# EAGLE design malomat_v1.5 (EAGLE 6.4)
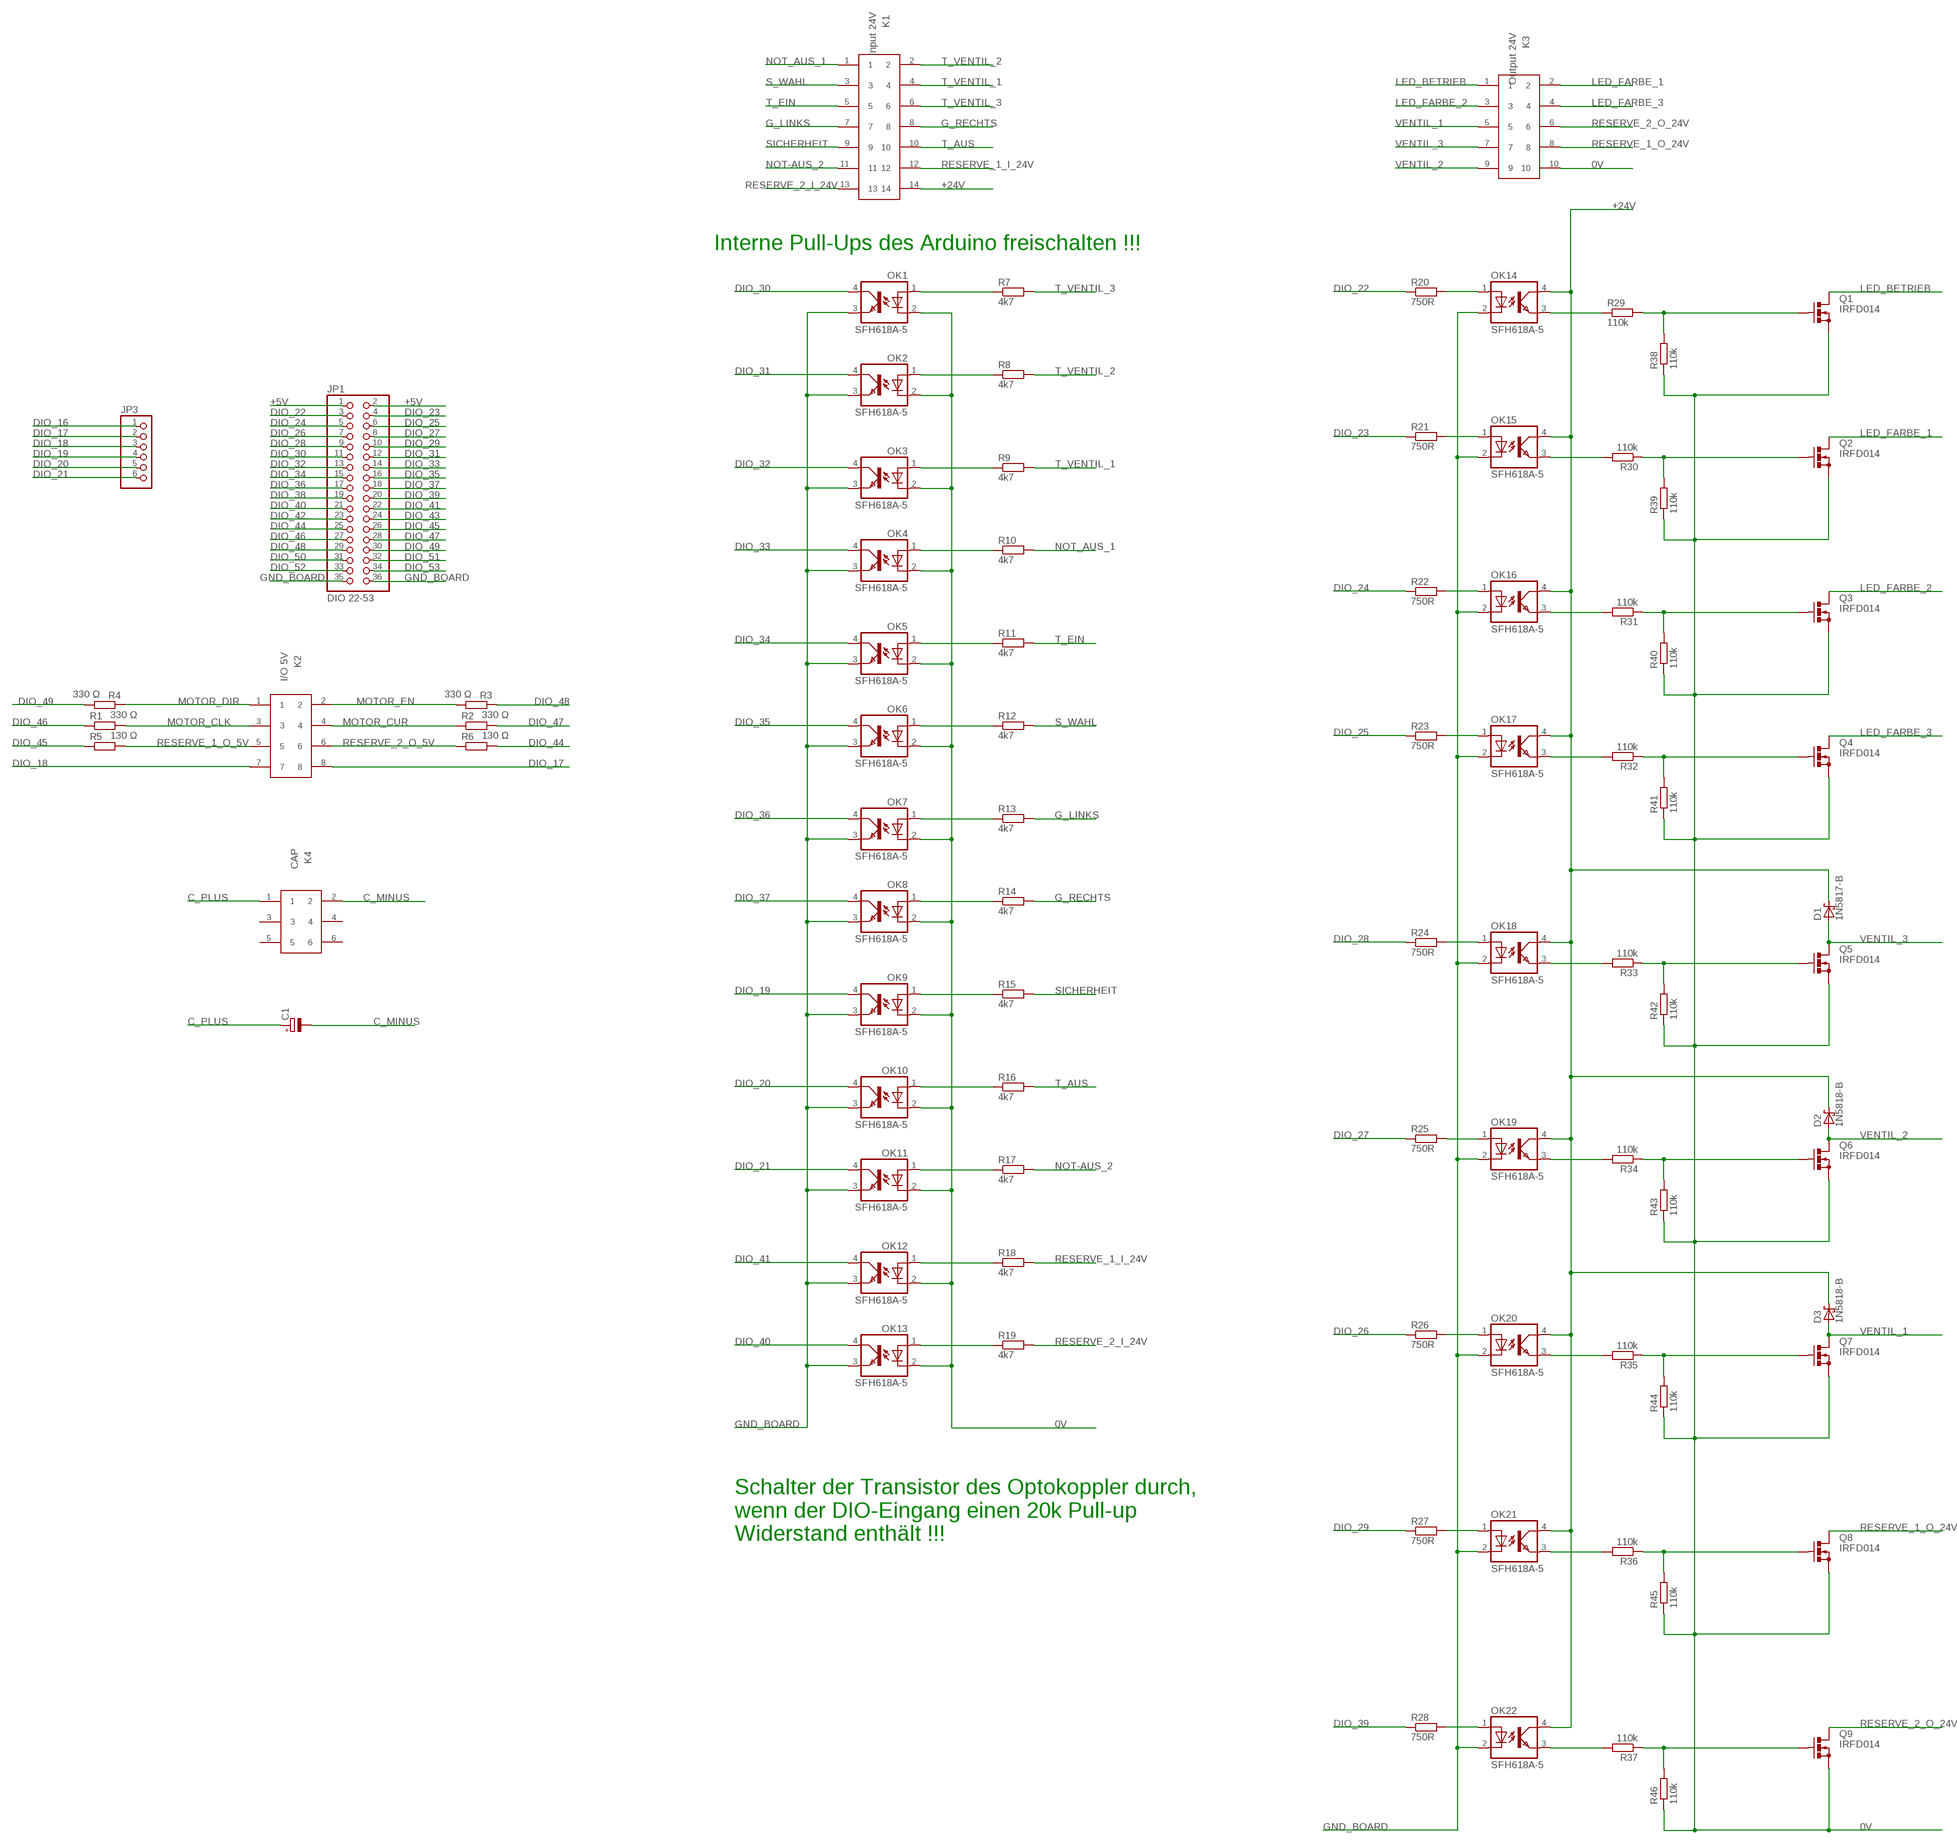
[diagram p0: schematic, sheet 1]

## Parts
C1  CPOL-EUE10-20  [EB20D]
D1  1N5817-B  [DO41-7.6]
D2  1N5818-B  [DO41-7.6]
D3  1N5818-B  [DO41-7.6]
JP1  DIO 22-53  PINHD-2X18  [2X18]
JP3  PINHD-1X6  [1X06]
K1  Input 24V  61201421621  [61201421621]
K2  I/O 5V  61200821621  [61200821621]
K3  Output 24V  61201021621  [61201021621]
K4  CAP  61200621621  [61200621621]
OK1  SFH618A-5  [DIP4]
OK2  SFH618A-5  [DIP4]
OK3  SFH618A-5  [DIP4]
OK4  SFH618A-5  [DIP4]
OK5  SFH618A-5  [DIP4]
OK6  SFH618A-5  [DIP4]
OK7  SFH618A-5  [DIP4]
OK8  SFH618A-5  [DIP4]
OK9  SFH618A-5  [DIP4]
OK10  SFH618A-5  [DIP4]
OK11  SFH618A-5  [DIP4]
OK12  SFH618A-5  [DIP4]
OK13  SFH618A-5  [DIP4]
OK14  SFH618A-5  [DIP4]
OK15  SFH618A-5  [DIP4]
OK16  SFH618A-5  [DIP4]
OK17  SFH618A-5  [DIP4]
OK18  SFH618A-5  [DIP4]
OK19  SFH618A-5  [DIP4]
OK20  SFH618A-5  [DIP4]
OK21  SFH618A-5  [DIP4]
OK22  SFH618A-5  [DIP4]
Q1  IRFD014  BS170  [C370-01]
Q2  IRFD014  BS170  [C370-01]
Q3  IRFD014  BS170  [C370-01]
Q4  IRFD014  BS170  [C370-01]
Q5  IRFD014  BS170  [C370-01]
Q6  IRFD014  BS170  [C370-01]
Q7  IRFD014  BS170  [C370-01]
Q8  IRFD014  BS170  [C370-01]
Q9  IRFD014  BS170  [C370-01]
R1  330 Ω  R-EU_0309/12  [0309/12]
R2  330 Ω  R-EU_0309/12  [0309/12]
R3  330 Ω  R-EU_0309/12  [0309/12]
R4  330 Ω  R-EU_0309/12  [0309/12]
R5  130 Ω  R-EU_0411/15  [0411/15]
R6  130 Ω  R-EU_0411/15  [0411/15]
R7  4k7  R-EU_0309/12  [0309/12]
R8  4k7  R-EU_0309/12  [0309/12]
R9  4k7  R-EU_0309/12  [0309/12]
R10  4k7  R-EU_0309/12  [0309/12]
R11  4k7  R-EU_0309/12  [0309/12]
R12  4k7  R-EU_0309/12  [0309/12]
R13  4k7  R-EU_0309/12  [0309/12]
R14  4k7  R-EU_0309/12  [0309/12]
R15  4k7  R-EU_0309/12  [0309/12]
R16  4k7  R-EU_0309/12  [0309/12]
R17  4k7  R-EU_0309/12  [0309/12]
R18  4k7  R-EU_0309/12  [0309/12]
R19  4k7  R-EU_0309/12  [0309/12]
R20  750R  R-EU_0204/7  [0204/7]
R21  750R  R-EU_0204/7  [0204/7]
R22  750R  R-EU_0204/7  [0204/7]
R23  750R  R-EU_0204/7  [0204/7]
R24  750R  R-EU_0204/7  [0204/7]
R25  750R  R-EU_0204/7  [0204/7]
R26  750R  R-EU_0204/7  [0204/7]
R27  750R  R-EU_0204/7  [0204/7]
R28  750R  R-EU_0204/7  [0204/7]
R29  110k  R-EU_0204/7  [0204/7]
R30  110k  R-EU_0204/7  [0204/7]
R31  110k  R-EU_0204/7  [0204/7]
R32  110k  R-EU_0204/7  [0204/7]
R33  110k  R-EU_0204/7  [0204/7]
R34  110k  R-EU_0204/7  [0204/7]
R35  110k  R-EU_0204/7  [0204/7]
R36  110k  R-EU_0204/7  [0204/7]
R37  110k  R-EU_0204/7  [0204/7]
R38  110k  R-EU_0204/7  [0204/7]
R39  110k  R-EU_0204/7  [0204/7]
R40  110k  R-EU_0204/7  [0204/7]
R41  110k  R-EU_0204/7  [0204/7]
R42  110k  R-EU_0204/7  [0204/7]
R43  110k  R-EU_0204/7  [0204/7]
R44  110k  R-EU_0204/7  [0204/7]
R45  110k  R-EU_0204/7  [0204/7]
R46  110k  R-EU_0204/7  [0204/7]

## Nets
0V: K3.10 OK1.2(C) OK2.2(C) OK3.2(C) OK4.2(C) OK5.2(C) OK6.2(C) OK7.2(C) OK8.2(C) OK9.2(C) OK10.2(C) OK11.2(C) OK12.2(C) OK13.2(C) Q1.S Q2.S Q3.S Q4.S Q5.S Q6.S Q7.S Q8.S Q9.S R38.1 R39.1 R40.1 R41.1 R42.1 R43.1 R44.1 R45.1 R46.1
+5V: JP1.1 JP1.2
+24V: D1.C D2.C D3.C K1.14 OK14.4(COL) OK15.4(COL) OK16.4(COL) OK17.4(COL) OK18.4(COL) OK19.4(COL) OK20.4(COL) OK21.4(COL) OK22.4(COL)
C_MINUS: C1.- K4.2
C_PLUS: C1.+ K4.1
DIO_16: JP3.1
DIO_17: JP3.2 K2.8
DIO_18: JP3.3 K2.7
DIO_19: JP3.4 OK9.4(COL)
DIO_20: JP3.5 OK10.4(COL)
DIO_21: JP3.6 OK11.4(COL)
DIO_22: JP1.3 R20.1
DIO_23: JP1.4 R21.1
DIO_24: JP1.5 R22.1
DIO_25: JP1.6 R23.1
DIO_26: JP1.7 R26.1
DIO_27: JP1.8 R25.1
DIO_28: JP1.9 R24.1
DIO_29: JP1.10 R27.1
DIO_30: JP1.11 OK1.4(COL)
DIO_31: JP1.12 OK2.4(COL)
DIO_32: JP1.13 OK3.4(COL)
DIO_33: JP1.14 OK4.4(COL)
DIO_34: JP1.15 OK5.4(COL)
DIO_35: JP1.16 OK6.4(COL)
DIO_36: JP1.17 OK7.4(COL)
DIO_37: JP1.18 OK8.4(COL)
DIO_38: JP1.19
DIO_39: JP1.20 R28.1
DIO_40: JP1.21 OK13.4(COL)
DIO_41: JP1.22 OK12.4(COL)
DIO_42: JP1.23
DIO_43: JP1.24
DIO_44: JP1.25 R6.2
DIO_45: JP1.26 R5.1
DIO_46: JP1.27 R1.1
DIO_47: JP1.28 R2.2
DIO_48: JP1.29 R3.1
DIO_49: JP1.30 R4.2
DIO_50: JP1.31
DIO_51: JP1.32
DIO_52: JP1.33
DIO_53: JP1.34
G_LINKS: K1.7 R13.2
G_RECHTS: K1.8 R14.2
GND_BOARD: JP1.35 JP1.36 OK1.3(EMIT) OK2.3(EMIT) OK3.3(EMIT) OK4.3(EMIT) OK5.3(EMIT) OK6.3(EMIT) OK7.3(EMIT) OK8.3(EMIT) OK9.3(EMIT) OK10.3(EMIT) OK11.3(EMIT) OK12.3(EMIT) OK13.3(EMIT) OK14.2(C) OK15.2(C) OK16.2(C) OK17.2(C) OK18.2(C) OK19.2(C) OK20.2(C) OK21.2(C) OK22.2(C)
LED_BETRIEB: K3.1 Q1.D
LED_FARBE_1: K3.2 Q2.D
LED_FARBE_2: K3.3 Q3.D
LED_FARBE_3: K3.4 Q4.D
MOTOR_CLK: K2.3 R1.2
MOTOR_CUR: K2.4 R2.1
MOTOR_DIR: K2.1 R4.1
MOTOR_EN: K2.2 R3.2
N$1: OK1.1(A) R7.1
N$2: OK2.1(A) R8.1
N$3: OK3.1(A) R9.1
N$4: OK22.1(A) R28.2
N$5: OK14.3(EMIT) R29.1
N$6: Q1.G R29.2 R38.2
N$7: OK4.1(A) R10.1
N$8: OK5.1(A) R11.1
N$9: OK6.1(A) R12.1
N$10: OK7.1(A) R13.1
N$13: OK21.1(A) R27.2
N$14: OK15.3(EMIT) R30.2
N$15: Q2.G R30.1 R39.2
N$16: OK8.1(A) R14.1
N$17: OK9.1(A) R15.1
N$18: OK10.1(A) R16.1
N$19: OK11.1(A) R17.1
N$20: OK12.1(A) R18.1
N$22: OK13.1(A) R19.1
N$23: OK20.1(A) R26.2
N$24: OK16.3(EMIT) R31.2
N$25: OK19.1(A) R25.2
N$26: Q3.G R31.1 R40.2
N$28: OK18.1(A) R24.2
N$29: OK17.1(A) R23.2
N$30: OK16.1(A) R22.2
N$31: OK15.1(A) R21.2
N$32: OK14.1(A) R20.2
N$35: OK17.3(EMIT) R32.2
N$36: Q4.G R32.1 R41.2
N$43: OK18.3(EMIT) R33.2
N$44: Q5.G R33.1 R42.2
N$50: OK19.3(EMIT) R34.2
N$51: Q6.G R34.1 R43.2
N$57: OK20.3(EMIT) R35.2
N$58: Q7.G R35.1 R44.2
N$64: OK21.3(EMIT) R36.2
N$65: Q8.G R36.1 R45.2
N$71: OK22.3(EMIT) R37.2
N$72: Q9.G R37.1 R46.2
NOT-AUS_2: K1.11 R17.2
NOT_AUS_1: K1.1 R10.2
RESERVE_1_I_24V: K1.12 R18.2
RESERVE_1_O_5V: K2.5 R5.2
RESERVE_1_O_24V: K3.8 Q8.D
RESERVE_2_I_24V: K1.13 R19.2
RESERVE_2_O_5V: K2.6 R6.1
RESERVE_2_O_24V: K3.6 Q9.D
S_WAHL: K1.3 R12.2
SICHERHEIT: K1.9 R15.2
T_AUS: K1.10 R16.2
T_EIN: K1.5 R11.2
T_VENTIL_1: K1.4 R9.2
T_VENTIL_2: K1.2 R8.2
T_VENTIL_3: K1.6 R7.2
VENTIL_1: D3.A K3.5 Q7.D
VENTIL_2: D2.A K3.9 Q6.D
VENTIL_3: D1.A K3.7 Q5.D
Unconnected: K4.3 K4.4 K4.5 K4.6

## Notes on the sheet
- Interne Pull-Ups des Arduino freischalten !!!
- Schalter der Transistor des Optokoppler durch, 
  wenn der DIO-Eingang einen 20k Pull-up 
  Widerstand enthält !!!

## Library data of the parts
C1 = resistor:CPOL-EU: POLARIZED CAPACITOR, European symbol
D1-D3 = diode:1N581*: 1.0A SCHOTTKY BARRIER RECTIFIER; MF: MULTICOMP; MPN: 1N4004; OC_FARNELL: 9565027
JP1 = pinhead:PINHD-2X18: PIN HEADER; MF: SAMTEC; MPN: TSW-118-07-F-D; OC_FARNELL: 2025187
JP3 = pinhead:PINHD-1X6: PIN HEADER
K1 = Wuerth_Elektronik_eiCan_05_Box_Header_IDC_Connectors_1_2:61201421621: WR-BHD 2.54mm Male Box Header, 14 Pins; MF: AMPHENOL; MPN: T821114A1R100CEU; OC_FARNELL: 2215292
K2 = Wuerth_Elektronik_eiCan_05_Box_Header_IDC_Connectors_1_2:61200821621: WR-BHD 2.54mm Male Box Header, 8 Pins; MF: AMPHENOL; MPN: T821108A1S100CEU; OC_FARNELL: 2215303
K3 = Wuerth_Elektronik_eiCan_05_Box_Header_IDC_Connectors_1_2:61201021621: WR-BHD 2.54mm Male Box Header, 10 Pins; MF: AMPHENOL; MPN: T821110A1S100CEU; OC_FARNELL: 2215304
K4 = Wuerth_Elektronik_eiCan_05_Box_Header_IDC_Connectors_1_2:61200621621: WR-BHD 2.54mm Male Box Header, 6 Pins
OK1-OK22 = optocoupler:SFH618?*: Optocoupler, Phototransistor Output, Low Input Current Source: Data sheet; MF: VISHAY/TELEFUNKEN; MPN: SFH618A-5; OC_FARNELL: 1469593; OC_NEWARK: 59K0259
Q1-Q9 = transistor-small-signal:BS170: N-CHANNEL MOS FET; OC_FARNELL: unknown
R1-R4 = resistor:R-EU_: RESISTOR, European symbol; MF: MULTICOMP; MPN: MF25 330R; OC_FARNELL: 9341730
R5 R6 = resistor:R-EU_: RESISTOR, European symbol; MF: MULTICOMP; MPN: MF50 130R; OC_FARNELL: 9339930
R7-R46 = rcl:R-EU_: RESISTOR, European symbol

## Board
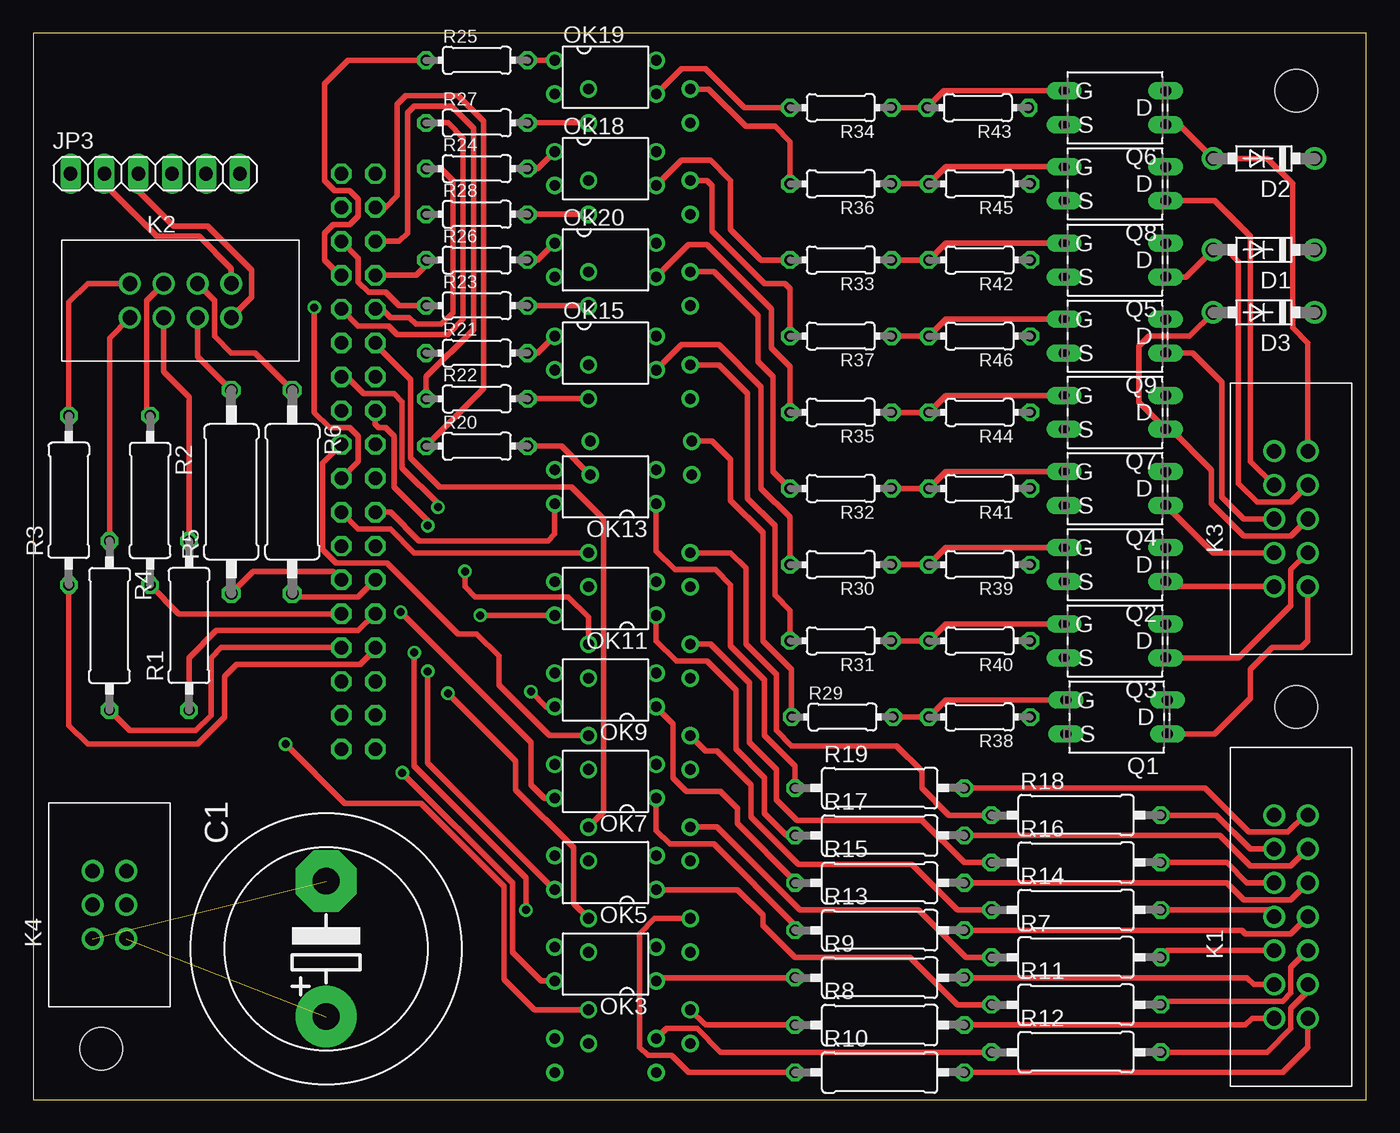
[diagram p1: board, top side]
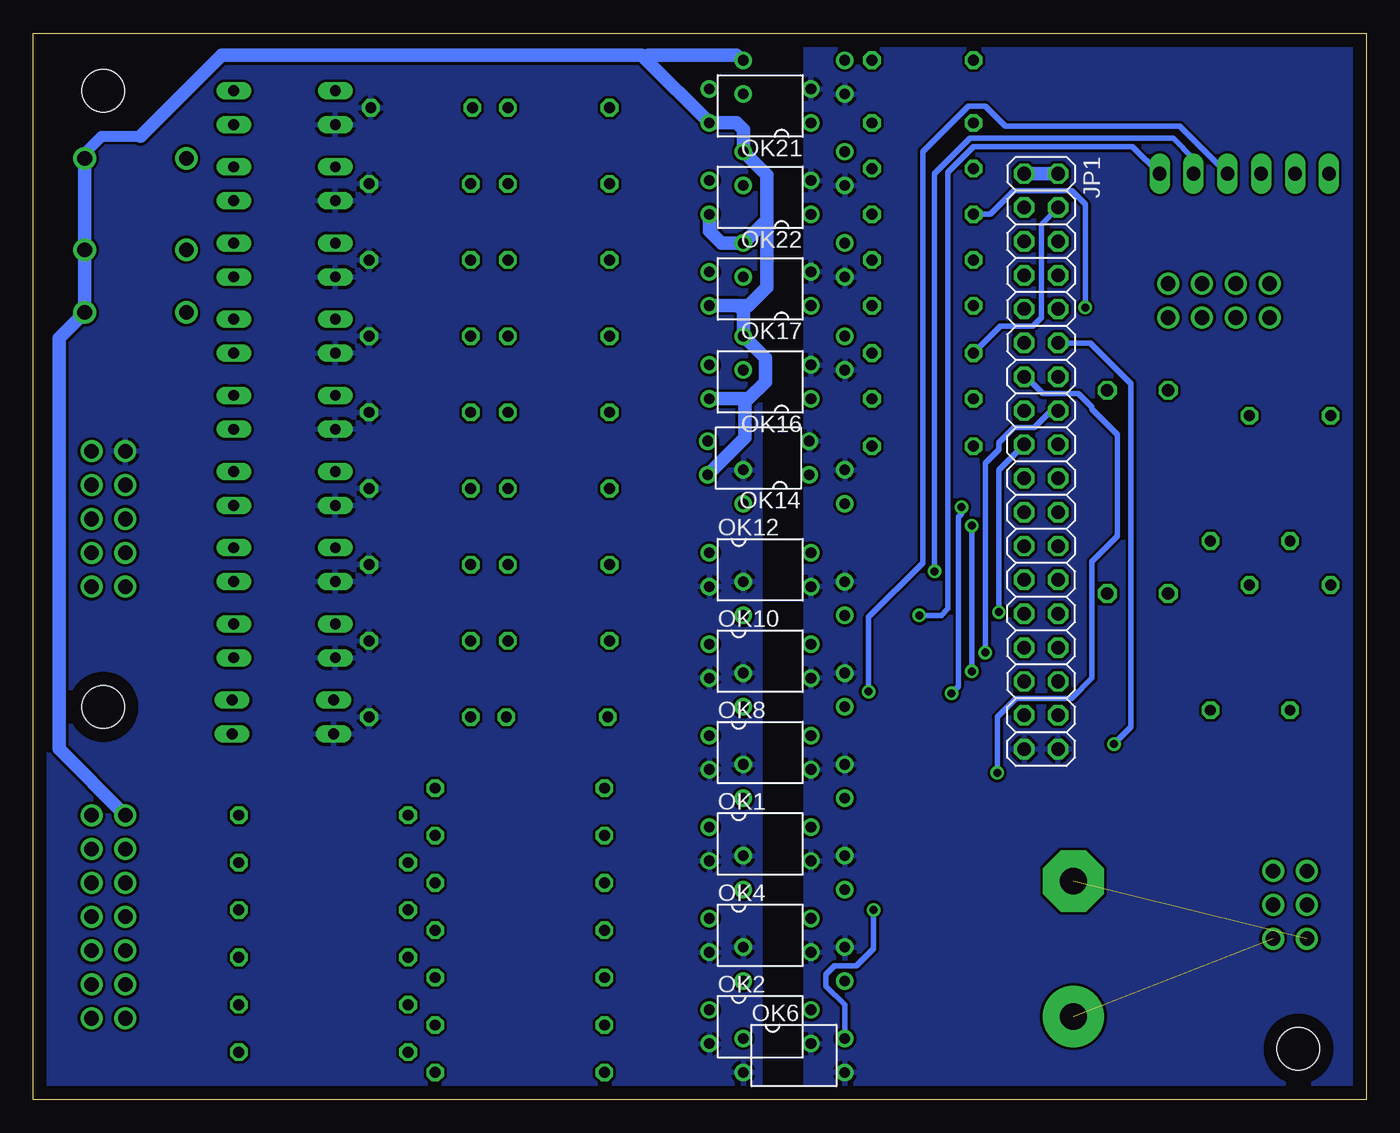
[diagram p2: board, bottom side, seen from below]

Size 100 x 80 mm. Coordinates in mm from the lower left corner, seen from the top.
Outline: 0,0 100,0 100,80 0,80 0,0
Copper layers (1*16): Top 0.035mm / dielectric 1.5mm / Bottom 0.035mm
Design rules "default": minimum track width 10mil, minimum drill 24mil, track to track 8mil, track to pad 8mil, pad to pad 8mil, via to via 8mil, smd to smd 8mil, copper to edge 40mil, drill to drill 8mil, minimum pad ring 10mil, minimum via ring 8mil, stop-mask expansion 4mil, vias tented up to drill 0mil, thermal gap 10mil
Holes 3.2 mm at 94.74,75.69 94.74,29.46 5.08,3.81

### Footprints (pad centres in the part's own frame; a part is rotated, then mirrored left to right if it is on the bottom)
EB20D = drill 2.007 pad 4.597: + -5.08,0 | drill 2.007 pad 4.597 octagon: - 5.08,0
DO41-7.6 = drill 1.1 pad 1.7: A 3.81,0; C -3.81,0
2X18 = drill 1.016 octagon: 1 -21.59,-1.27; 2 -21.59,1.27; 3 -19.05,-1.27; 4 -19.05,1.27; 5 -16.51,-1.27; 6 -16.51,1.27; 7 -13.97,-1.27; 8 -13.97,1.27; 9 -11.43,-1.27; 10 -11.43,1.27; 11 -8.89,-1.27; 12 -8.89,1.27; 13 -6.35,-1.27; 14 -6.35,1.27; 15 -3.81,-1.27; 16 -3.81,1.27; 17 -1.27,-1.27; 18 -1.27,1.27; 19 1.27,-1.27; 20 1.27,1.27; 21 3.81,-1.27; 22 3.81,1.27; 23 6.35,-1.27; 24 6.35,1.27; 25 8.89,-1.27; 26 8.89,1.27; 27 11.43,-1.27; 28 11.43,1.27; 29 13.97,-1.27; 30 13.97,1.27; 31 16.51,-1.27; 32 16.51,1.27; 33 19.05,-1.27; 34 19.05,1.27; 35 21.59,-1.27; 36 21.59,1.27
1X06 = drill 1.016 long: 1 -6.35,0; 2 -3.81,0; 3 -1.27,0; 4 1.27,0; 5 3.81,0; 6 6.35,0
61201421621 = drill 1.1: 1 -2.54,-1.27; 2 -2.54,1.27; 3 0,-1.27; 4 0,1.27; 5 2.54,-1.27; 6 2.54,1.27; 7 5.08,-1.27; 8 5.08,1.27; 9 7.62,-1.27; 10 7.62,1.27; 11 10.16,-1.27; 12 10.16,1.27; 13 12.7,-1.27; 14 12.7,1.27
61200821621 = drill 1.1: 1 -2.54,-1.27; 2 -2.54,1.27; 3 0,-1.27; 4 0,1.27; 5 2.54,-1.27; 6 2.54,1.27; 7 5.08,-1.27; 8 5.08,1.27
61201021621 = drill 1.1: 1 -2.54,-1.27; 2 -2.54,1.27; 3 0,-1.27; 4 0,1.27; 5 2.54,-1.27; 6 2.54,1.27; 7 5.08,-1.27; 8 5.08,1.27; 9 7.62,-1.27; 10 7.62,1.27
61200621621 = drill 1.1: 1 -2.54,-1.27; 2 -2.54,1.27; 3 0,-1.27; 4 0,1.27; 5 2.54,-1.27; 6 2.54,1.27
DIP4 = drill 0.8: 1 -1.27,-3.81; 2 1.27,-3.81; 3 1.27,3.81; 4 -1.27,3.81
C370-01 = drill 0.813 long: D -3.81,1.27; D1 -3.81,-1.27; G 3.81,-1.27; S 3.81,1.27
0309/12 = drill 0.813 octagon: 1 -6.35,0; 2 6.35,0
0411/15 = drill 0.914 octagon: 1 -7.62,0; 2 7.62,0
0204/7 = drill 0.813 octagon: 1 -3.81,0; 2 3.81,0

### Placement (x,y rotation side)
C1  21.97,11.3 90 top
D1  92.33,63.75 180 top
D2  92.33,70.61 180 top
D3  92.33,59.05 180 top
JP1  24.38,47.88 270 bottom
JP3  9.14,69.47 0 top
K1  94.36,8.64 90 top
K2  9.78,59.94 0 top
K3  94.36,41.02 90 top
K4  5.71,14.61 90 top
OK1  45.47,19.18 270 bottom
OK2  45.47,5.46 270 bottom
OK3  42.93,10.16 90 top
OK4  45.47,12.32 270 bottom
OK5  42.93,17.02 90 top
OK6  42.93,3.3 270 bottom
OK7  42.93,23.88 90 top
OK8  45.47,26.04 270 bottom
OK9  42.93,30.73 90 top
OK10  45.47,32.89 270 bottom
OK11  42.93,37.59 90 top
OK12  45.47,39.75 270 bottom
OK13  42.93,45.97 90 top
OK14  45.59,48.13 90 bottom
OK15  42.93,56.01 270 top
OK16  45.47,53.85 90 bottom
OK17  45.47,60.83 90 bottom
OK18  42.93,69.85 270 top
OK19  42.93,76.71 270 top
OK20  42.93,62.99 270 top
OK21  45.47,74.55 90 bottom
OK22  45.47,67.69 90 bottom
Q1  81.28,28.7 180 top
Q2  81.15,40.13 180 top
Q3  81.15,34.42 180 top
Q4  81.15,45.85 180 top
Q5  81.15,62.99 180 top
Q6  81.15,74.42 180 top
Q7  81.15,51.56 180 top
Q8  81.15,68.71 180 top
Q9  81.15,57.28 180 top
R1  11.68,35.56 90 top
R2  8.76,44.96 270 top
R3  2.67,44.96 90 top
R4  5.71,35.56 270 top
R5  14.86,45.59 90 top
R6  19.43,45.59 270 top
R7  78.23,10.67 0 top
R8  63.5,5.59 0 top
R9  63.5,9.14 0 top
R10  63.5,2.03 0 top
R11  78.23,7.11 0 top
R12  78.23,3.56 0 top
R13  63.5,12.7 0 top
R14  78.23,14.22 0 top
R15  63.5,16.26 0 top
R16  78.23,17.78 0 top
R17  63.5,19.81 0 top
R18  78.23,21.34 0 top
R19  63.5,23.37 0 top
R20  33.27,49.02 0 top
R21  33.27,56.01 0 top
R22  33.27,52.58 0 top
R23  33.27,59.56 0 top
R24  33.27,69.85 0 top
R25  33.27,77.98 0 top
R26  33.27,62.99 0 top
R27  33.27,73.28 0 top
R28  33.27,66.42 0 top
R29  60.71,28.7 0 top
R30  60.58,40.13 180 top
R31  60.58,34.42 180 top
R32  60.58,45.85 180 top
R33  60.58,62.99 180 top
R34  60.58,74.42 180 top
R35  60.58,51.56 180 top
R36  60.58,68.71 180 top
R37  60.58,57.28 180 top
R38  70.99,28.7 180 top
R39  70.99,40.13 180 top
R40  70.99,34.42 180 top
R41  70.99,45.85 180 top
R42  70.99,62.99 180 top
R43  70.87,74.42 180 top
R44  70.99,51.56 180 top
R45  70.99,68.71 180 top
R46  70.99,57.28 180 top

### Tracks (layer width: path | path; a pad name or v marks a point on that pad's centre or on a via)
0V
  pour Bottom: 99.95,0 45.47,-0.13 45.47,80.01 99.95,80.14
+5V
  Bottom 1.016: JP1.2 JP1.1
+24V
  Bottom 0.813: D3.C 96.14,70.99 94.87,72.26 91.95,72.26
  Bottom 1.016: K1.14 98.04,26.29 98.04,57.15 D3.C D1.C D2.C | 91.95,72.26 85.85,78.36 54.36,78.36 54.1,78.11 | 54.1,78.11 OK21.4 47.24,73.28 46.74,72.77 OK18.4 44.96,69.34 44.96,66.04 45.09,65.91 | OK19.4 46.86,77.98 47.24,78.36 53.85,78.36 54.1,78.11 | 45.09,65.91 OK20.4 48.39,64.26 49.28,65.15 OK22.4 | 47.12,59.56 46.74,59.18 OK15.4 45.09,55.63 45.09,53.85 46.35,52.58 46.61,52.58 | 47.12,59.56 OK17.4 | 47.12,59.56 46.35,59.56 44.96,60.96 44.96,65.79 45.09,65.91 | OK16.4 46.61,52.58 | OK14.4 46.61,49.66 46.61,52.58
C_MINUS  (1 unrouted)
C_PLUS  (1 unrouted)
DIO_17
  Top 0.406: JP3.2 5.33,68.71 9.27,64.77 12.45,64.77 14.86,62.36 K2.8
DIO_18
  Top 0.406: JP3.3 7.87,68.2 10.54,65.53 13.08,65.53 16.38,62.23 16.38,60.2 K2.7
DIO_19  (via drill 0.6)
  Top 0.406: OK9.4 38.48,29.46 v37.34,30.61
  Bottom 0.406: v37.34,30.61 37.34,36.2 33.27,40.26 33.27,71.12 29.84,74.55 28.57,74.55 27.05,73.03 13.97,73.03 JP3.4
DIO_20  (via drill 0.6)
  Top 0.406: v32.38,39.62 32.38,38.48 33.15,37.72 40.13,37.72 41.66,36.2 OK10.4
  Bottom 0.406: v32.38,39.62 32.38,69.47 29.72,72.14 14.48,72.14 12.95,70.61 JP3.5
DIO_21  (via drill 0.6)
  Top 0.406: OK11.4 v33.53,36.32
  Bottom 0.406: JP3.6 17.53,71.5 29.46,71.5 31.37,69.6 31.37,36.83 31.88,36.32 v33.53,36.32
DIO_22
  Top 0.406: JP1.3 26.42,66.93 27.3,67.82 27.3,74.68 27.94,75.31 31.88,75.31 33.78,73.41 33.78,53.34 R20.1
DIO_23
  Bottom 0.406: JP1.4 24.38,65.66 24.38,58.67 25.02,58.04 27.43,58.04 R21.1
DIO_24
  Top 0.406: JP1.5 27.43,64.39 28.07,65.02 28.07,74.04 28.57,74.55 31.37,74.55 33.02,72.9 33.02,57.78 29.46,54.23 R22.1
DIO_25
  Top 0.406: R23.1 27.43,59.56 26.42,60.58 25.15,60.58 24.38,61.34 24.38,63.12 JP1.6
DIO_26
  Top 0.406: R26.1 29.46,62.61 28.7,61.85 JP1.7
DIO_27
  Top 0.406: JP1.8 22.99,61.85 21.84,62.99 21.84,65.02 22.48,65.66 23.75,65.66 24.38,66.29 24.38,67.56 23.75,68.2 22.61,68.2 21.84,68.96 21.84,76.2 23.62,77.98 R25.1
DIO_28
  Top 0.406: JP1.9 26.16,59.31 26.8,58.67 28.19,58.67 28.7,58.17 30.61,58.17 31.5,59.05 31.5,68.96 30.61,69.85 R24.1
DIO_29
  Top 0.406: 29.59,73.28 R27.1 31.11,73.28 32.26,72.14 32.26,58.55 31.11,57.4 27.3,57.4 26.67,58.04 24.38,58.04 JP1.10
DIO_30
  Top 0.254: 42.65,21.51 41.76,20.62 OK1.4
  Top 0.406: JP1.11 25.65,56.67 28.32,54 28.32,48.13 30.48,45.97 40.39,45.97 42.8,43.56 42.8,21.59 OK1.4
DIO_31  (via drill 0.6)
  Top 0.406: v18.92,26.67 23.37,22.23 29.08,22.23 35.31,16 35.31,9.02 37.59,6.73 OK2.4
  Bottom 0.406: JP1.12 20.7,56.77 17.65,53.72 17.65,27.94 v18.92,26.67
DIO_32  (via drill 0.6)
  Top 0.406: v27.69,24.51 35.94,16.26 35.94,11.05 38.1,8.89 OK3.4
  Bottom 0.406: JP1.13 25.53,54.23 24.26,52.96 21.59,52.96 20.57,51.94 20.57,51.82 18.67,49.91 18.67,42.29 20.57,40.39 20.57,31.62 22.1,30.1 26.29,30.1 27.69,28.7 v27.69,24.51
DIO_33  (via drill 0.6)
  Top 0.406: OK4.4 40.51,14.73 40.51,18.92 36.2,23.24 36.2,25.4 v31.11,30.48 | JP1.14 23.5,54.23 24.77,52.96 27.05,52.96 27.69,52.32 27.69,47.37 30.35,44.7 v30.35,44.45
  Bottom 0.406: v31.11,30.48 30.61,30.99 30.61,43.69 30.35,43.94 v30.35,44.45
DIO_34  (via drill 0.6)
  Top 0.406: JP1.15 25.65,50.67 25.91,50.42 26.42,50.42 27.05,49.78 27.05,45.97 29.59,43.43 v29.59,43.05 | v29.59,32.13 29.59,25.27 OK5.4
  Bottom 0.406: v29.59,43.05 v29.59,32.13
DIO_35  (via drill 0.6)
  Top 0.406: v36.96,14.22 36.96,16.64 28.57,25.02 v28.57,33.53
  Bottom 0.406: 38.99,4.57 OK6.4 39.12,7.11 40.51,8.51 40.51,9.4 39.88,10.03 38.23,10.03 36.96,11.3 v36.96,14.22 | v28.57,33.53 28.57,47.75 27.56,48.77 27.56,49.28 26.42,50.42 24.89,50.42 23.62,51.69 JP1.16
DIO_36  (via drill 0.6)
  Top 0.406: OK7.4 38.35,22.61 37.34,23.62 37.34,26.8 v27.56,36.58
  Bottom 0.406: v27.56,36.58 27.56,47.24 JP1.17
DIO_37
  Top 0.406: OK8.4 38.73,27.3 34.92,31.11 34.92,33.27 33.27,34.92 31.88,34.92 26.54,40.26 22.73,40.26 21.72,41.27 21.72,47.75 JP1.18
DIO_39  (via drill 0.6)
  Top 0.406: v21.08,59.44 21.08,51.56 22.23,50.42 23.75,50.42 24.38,49.78 24.38,47.88 JP1.20
  Bottom 0.406: R28.1 28.19,66.42 26.42,68.2 22.1,68.2 21.08,67.18 v21.08,59.44
DIO_40
  Top 0.406: JP1.21 26.8,44.07 28.96,41.91 38.61,41.91 39.12,42.42 OK13.4
DIO_41
  Top 0.406: OK12.4 28.57,41.02 26.8,42.8 24.38,42.8 JP1.22
DIO_44
  Top 0.406: JP1.25 24.38,37.72 19.68,37.72 R6.2
DIO_45
  Top 0.406: R5.1 16.51,39.62 22.48,39.62 JP1.26
DIO_46
  Top 0.406: JP1.27 24.38,35.18 13.72,35.18 11.68,33.15 R1.1
DIO_47
  Top 0.406: JP1.28 10.92,36.45 R2.2
DIO_48
  Top 0.406: JP1.29 25.65,33.78 24.51,32.64 15.24,32.64 14.35,31.75 14.35,28.7 12.32,26.67 4.06,26.67 2.67,28.07 R3.1
DIO_49
  Top 0.406: JP1.30 14.1,33.91 13.34,33.15 13.34,28.83 12.19,27.69 7.24,27.69 R4.2
G_LINKS
  Top 0.406: K1.7 94.36,12.45 90.93,12.45 90.68,12.7 R13.2
G_RECHTS
  Top 0.406: R14.2 92.58,14.22 K1.8
GND_BOARD
  pour Bottom: 0,0 42.04,0 42.04,80.01 0,80.01
LED_BETRIEB
  Top 0.406: K3.1 95.63,34.42 95.12,33.91 92.96,33.91 91.31,32.26 91.31,30.1 88.65,27.43 Q1.D
LED_FARBE_1
  Top 0.406: K3.2 85.34,38.48 Q2.D
LED_FARBE_2
  Top 0.406: Q3.D 90.42,33.15 94.36,37.08 94.36,39.75 K3.3
LED_FARBE_3
  Top 0.406: K3.4 88.52,41.02 Q4.D
MOTOR_CLK
  Top 0.406: K2.3 9.78,54.61 11.68,52.7 R1.2
MOTOR_CUR
  Top 0.406: K2.4 8.51,59.94 8.51,51.56 R2.1
MOTOR_DIR
  Top 0.406: K2.1 5.71,57.15 R4.1
MOTOR_EN
  Top 0.406: K2.2 4.06,61.21 2.67,59.82 R3.2
N$1
  Top 0.406: R7.1 69.98,10.67 66.42,14.22 57.53,14.22 51.31,20.45 OK1.1
N$2
  Top 0.406: R8.1 50.42,5.59 OK2.1
N$3
  Top 0.406: R9.1 46.99,9.14 OK3.1
N$4
  Top 0.406: R28.2 OK22.1
N$5
  Top 0.406: R29.1 56.9,32.26 54.74,34.42 54.74,42.55 52.32,44.96 52.32,48.01 50.93,49.4 OK14.3
N$6
  Top 0.406: Q1.G 68.45,29.97 R38.2 R29.2
N$7
  Top 0.406: R10.1 49.15,2.03 47.88,3.3 46.1,3.3 45.47,3.94 45.47,12.45 46.61,13.59 OK4.1
N$8
  Top 0.406: R11.1 69.34,7.11 65.79,10.67 57.15,10.67 54.74,13.08 54.74,13.84 52.83,15.75 OK5.1
N$9
  Top 0.406: R12.1 51.56,3.56 49.78,5.33 47.5,5.33 OK6.1
N$10
  Top 0.406: R13.1 57.15,13.08 51.05,19.18 47.75,19.18 46.74,20.19 OK7.1
N$13
  Top 0.406: R27.2 OK21.1
N$14
  Top 0.406: R30.2 56.77,43.69 54.61,45.85 54.61,53.47 51.44,56.64 48.64,56.64 OK15.3
N$15
  Top 0.406: Q2.G 68.45,41.4 R39.2 | R39.2 67.31,40.13 | R39.2 R30.1
N$16
  Top 0.406: R14.1 69.34,14.22 65.91,17.65 57.4,17.65 53.85,21.21 53.85,23.62 51.31,26.16 50.42,26.16 OK8.1
N$17
  Top 0.406: R15.1 57.15,16.38 52.83,20.7 52.83,21.84 51.56,23.11 49.02,23.11 48.01,24.13 48.01,28.19 OK9.1
N$18
  Top 0.406: R16.1 69.85,17.78 66.67,20.95 57.28,20.95 55.75,22.48 55.75,24.77 53.72,26.8 53.72,31.24 50.8,34.16 OK10.1
N$19
  Top 0.406: R17.1 56.52,19.81 54.86,21.46 54.86,24.13 52.7,26.29 52.7,30.73 50.55,32.89 48.26,32.89 46.74,34.42 OK11.1
N$20
  Top 0.406: R18.1 68.71,21.34 66.67,23.37 66.67,24.64 64.77,26.54 56.9,26.54 55.75,27.69 55.75,31.88 53.47,34.16 53.47,39.88 52.32,41.02 OK12.1
N$22
  Top 0.406: R19.1 57.15,25.02 54.86,27.3 54.86,31.5 52.32,34.04 52.32,38.61 51.18,39.75 48.13,39.75 46.74,41.15 OK13.1
N$23
  Top 0.406: R26.2 37.85,62.99 OK20.1
N$24
  Top 0.406: OK16.3 51.44,55.12 53.59,52.96 53.59,45.09 55.63,43.05 55.63,37.85 56.77,36.7 R31.2
N$25
  Top 0.406: R25.2 OK19.1
N$26
  Top 0.406: Q3.G 68.45,35.69 R40.2 R31.1
N$28
  Top 0.406: R24.2 37.85,69.85 OK18.1
N$29
  Top 0.406: R23.2 OK17.1
N$30
  Top 0.406: R22.2 OK16.1
N$31
  Top 0.406: R21.2 37.85,56.01 OK15.1
N$32
  Top 0.406: R20.2 39.62,49.02 OK14.1
N$35
  Top 0.406: OK17.3 51.05,62.1 54.36,58.8 54.36,55.37 55.5,54.23 55.5,47.12 R32.2
N$36
  Top 0.406: Q4.G 68.45,47.12 R41.2 R32.1
N$43
  Top 0.406: R33.2 54.61,62.99 52.32,65.28 52.32,68.96 50.8,70.48 48.64,70.48 OK18.3
N$44
  Top 0.406: Q5.G 68.45,64.26 R42.2 R33.1
N$50
  Top 0.406: R34.2 53.34,74.42 50.42,77.34 48.64,77.34 OK19.3
N$51
  Top 0.406: Q6.G 68.33,75.69 R43.2 R34.1
N$57
  Top 0.406: R35.2 56.77,54.99 55.37,56.39 55.37,59.31 50.55,64.14 49.15,64.14 OK20.3
N$58
  Top 0.406: Q7.G 68.45,52.83 R44.2 R35.1
N$64
  Top 0.406: OK21.3 50.67,75.82 53.47,73.03 55.63,73.03 56.77,71.88 R36.2
N$65
  Top 0.406: Q8.G 68.45,69.98 R45.2 R36.1
N$71
  Top 0.406: OK22.3 50.55,68.96 50.93,68.58 50.93,65.15 54.86,61.21 56.39,61.21 56.77,60.83 R37.2
N$72
  Top 0.406: Q9.G 68.45,58.55 R46.2 R37.1
NOT-AUS_2
  Top 0.406: K1.11 94.36,17.53 91.31,17.53 89.03,19.81 R17.2
NOT_AUS_1
  Top 0.406: R10.2 93.73,2.03 95.63,3.94 K1.1
RESERVE_1_I_24V
  Top 0.406: R18.2 88.77,21.34 91.31,18.8 K1.12
RESERVE_1_O_5V
  Top 0.406: K2.5 12.32,55.75 R5.2
RESERVE_1_O_24V
  Top 0.406: Q8.D 88.65,67.44 91.31,64.77 91.31,47.88 K3.8
RESERVE_2_I_24V
  Top 0.406: K1.13 95.38,21.34 94.11,20.07 91.19,20.07 87.88,23.37 R19.2
RESERVE_2_O_5V
  Top 0.406: K2.6 13.59,59.94 13.59,57.28 14.86,56.01 16.64,56.01 R6.1
RESERVE_2_O_24V
  Top 0.406: Q9.D 87,56.01 89.15,53.85 89.15,45.21 90.81,43.56 K3.6
S_WAHL
  Top 0.406: K1.3 95.63,8.13 94.36,6.86 94.36,5.33 92.58,3.56 R12.2
SICHERHEIT
  Top 0.406: K1.9 94.36,14.99 90.81,14.99 89.53,16.26 R15.2
T_AUS
  Top 0.406: R16.2 89.53,17.78 91.06,16.26 K1.10
T_EIN
  Top 0.406: K1.5 94.36,9.91 94.36,8 93.73,7.37 84.84,7.37 R11.2
T_VENTIL_1
  Top 0.406: K1.4 91.57,8.64 91.06,9.14 R9.2
T_VENTIL_2
  Top 0.406: K1.2 91.44,6.1 90.93,5.59 R8.2
T_VENTIL_3
  Top 0.406: K1.6 85.09,11.18 R7.2
VENTIL_1
  Top 0.406: K3.5 94.36,42.29 90.81,42.29 88.39,44.7 88.39,47.24 85.34,50.29 Q7.D 82.93,52.32 82.93,56.52 83.69,57.28 86.74,57.28 D3.A
VENTIL_2
  Top 0.406: Q6.D 85.98,73.15 D2.A 92.58,70.61 94.49,68.71 94.49,57.91 95.63,56.77 K3.9
VENTIL_3
  Top 0.406: Q5.D 86.49,61.72 D1.A 89.53,63.75 90.42,62.87 90.42,46.23 91.82,44.83 94.36,44.83 K3.7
